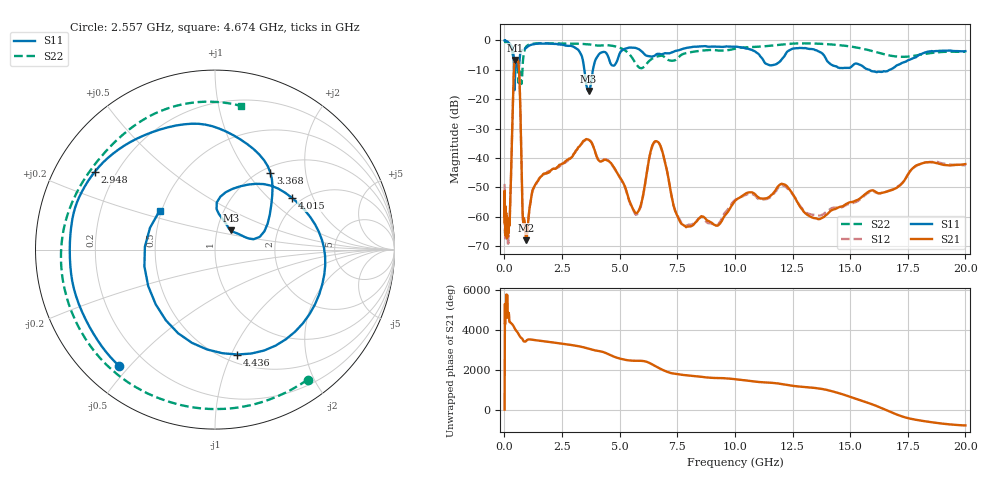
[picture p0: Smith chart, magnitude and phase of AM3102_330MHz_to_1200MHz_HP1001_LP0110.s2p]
! Date/Time: Tue, Sep 11, 2018 5:18 PM
! Network Analyzer: Agilent Technologies E8362B Rev: A.07.50.63
! Sweep from 0.010 to 20.000 GHz, 1601 Points, Sweep Type: LOG
! Power Supply: 4.949 V, 0.001 A
# Hz S DB R 50
!freq MagS11 AngS11 MagS21 AngS21 MagS12 AngS12 MagS22 AngS22
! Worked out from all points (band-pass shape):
!   1601 points, 10 MHz to 20 GHz, reference 50 ohm
!   highest |S21| = -6.61 dB at 464.5 MHz (marker M1); lowest = -68.0 dB at 947.3 MHz (marker M2)
!   |S21| within 3 dB of the highest: 415.9 MHz to 631.9 MHz (216 MHz wide, 41.2 % of centre)
!   lowest |S11| = -17.2 dB at 3.651 GHz (marker M3), VSWR 1.32, Z = 58.1 + j12.6 ohm
!   |S11| at or under -10 dB: 417.8 MHz to 471.1 MHz (53.29 MHz wide, 12 % of centre); 3.471 GHz to 3.841 GHz (370.7 MHz wide, 10.1 % of centre); 15.84 GHz to 16.71 GHz (872.2 MHz wide, 5.36 % of centre)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
!   |S22| runs from -14.8 to -0.2 dB; largest |S21 - S12| = 0.0079
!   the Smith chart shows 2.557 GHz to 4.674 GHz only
!   S11 on the Smith chart (normalised r, x): 2.557 GHz: 0.11, -0.47; 2.948 GHz: 0.12, +0.29; 3.368 GHz: 1.09, +1.30; 4.015 GHz: 1.80, +1.41; 4.436 GHz: 0.58, -1.06; 4.674 GHz: 0.49, +0.25
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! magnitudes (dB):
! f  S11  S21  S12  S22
! 10 MHz  0.0  -59.3  -49.2  -0.2
! 35.55 MHz  0.0  -64.7  -64.8  -0.3
! 126.4 MHz  -0.4  -65.8  -63.9  -0.8
! 234.4 MHz  -1.1  -60.7  -60.6  -1.4
! 447.2 MHz  -16.7  -6.8  -6.9  -7.6
! 464.5 MHz  -11.8  -6.6  -6.7  -7.0
! 632.6 MHz  -8.9  -9.7  -9.7  -13.7
! 794.6 MHz  -3.3  -59.4  -60.2  -8.3
! 947.3 MHz  -2.5  -68.0  -68.0  -2.1
! 1.59 GHz  -1.0  -46.3  -46.2  -1.0
! 2.557 GHz  -1.5  -41.9  -41.9  -1.0
! 2.948 GHz  -2.0  -39.5  -39.2  -1.0
! 3.368 GHz  -5.5  -34.9  -35.0  -1.2
! 3.651 GHz  -17.2  -33.8  -33.5  -1.3
! 4.015 GHz  -5.7  -39.7  -39.6  -1.7
! 4.436 GHz  -4.5  -40.7  -40.6  -1.6
! 4.674 GHz  -8.5  -42.3  -42.4  -1.8
! 5.652 GHz  -2.5  -58.3  -58.8  -7.2
! 6.58 GHz  -4.8  -34.3  -34.4  -5.5
! 7.92 GHz  -2.5  -63.4  -62.9  -4.2
! 13.68 GHz  -3.9  -60.8  -59.6  -1.1
! 20 GHz  -3.6  -42.1  -42.5  -3.9
